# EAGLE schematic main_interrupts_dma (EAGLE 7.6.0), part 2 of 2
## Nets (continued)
Unconnected: IC1.1(CLR) IC1.11(CLK) IC2.1(A:G) IC2.2(A:A1) IC2.4(A:A2) IC2.6(A:A3) IC2.8(A:A4) IC2.12(A:Y4) IC2.14(A:Y3) IC2.16(A:Y2) IC2.18(A:Y1) IC3.1(A:G) IC3.2(A:A1) IC3.4(A:A2) IC3.6(A:A3) IC3.8(A:A4) IC3.12(A:Y4) IC3.14(A:Y3) IC3.16(A:Y2) IC3.18(A:Y1) IC4.11(CLK) IC5.11(CLK) IC6.11(CLK) IC10.3(B:Y4) IC10.17(B:A4) IC11.3(B:Y4) IC11.5(B:Y3) IC11.7(B:Y2) IC11.9(B:Y1) IC11.11(B:A1) IC11.13(B:A2) IC11.15(B:A3) IC11.17(B:A4) IC11.19(B:G) IC12.3(B:Y4) IC12.5(B:Y3) IC12.7(B:Y2) IC12.9(B:Y1) IC12.11(B:A1) IC12.13(B:A2) IC12.15(B:A3) IC12.17(B:A4) IC12.19(B:G) IC13.3(B:Y4) IC13.5(B:Y3) IC13.7(B:Y2) IC13.9(B:Y1) IC13.11(B:A1) IC13.13(B:A2) IC13.15(B:A3) IC13.17(B:A4) IC13.19(B:G) IC14.14(A=B) IC14.15(P) IC14.17(G) IC15.14(A=B) IC15.15(P) IC15.17(G) IC16.11(CLK) IC17.11(CLK) IC18.1(A:I0) IC18.2(A:I1) IC18.3(A:O) IC18.8(C:O) IC18.9(C:I0) IC18.10(C:I1) IC18.11(D:O) IC18.12(D:I0) IC18.13(D:I1) IC19.2(A:A1) IC19.4(A:A2) IC19.6(A:A3) IC19.8(A:A4) IC19.11(B:A1) IC19.13(B:A2) IC19.15(B:A3) IC19.17(B:A4) IC20.11(CLK) IC21.11(CLK) IC24.1(A:G) IC24.2(A:A1) IC24.4(A:A2) IC24.6(A:A3) IC24.8(A:A4) IC24.12(A:Y4) IC24.14(A:Y3) IC24.16(A:Y2) IC24.18(A:Y1) IC24.19(B:G) IC25.1(A:G) IC25.2(A:A1) IC25.4(A:A2) IC25.6(A:A3) IC25.8(A:A4) IC25.12(A:Y4) IC25.14(A:Y3) IC25.16(A:Y2) IC25.18(A:Y1) IC25.19(B:G) IC26.1(A:G) IC26.2(A:A1) IC26.4(A:A2) IC26.6(A:A3) IC26.8(A:A4) IC26.12(A:Y4) IC26.14(A:Y3) IC26.16(A:Y2) IC26.18(A:Y1) IC26.19(B:G) IC27.1(A:G) IC27.2(A:A1) IC27.4(A:A2) IC27.6(A:A3) IC27.8(A:A4) IC27.12(A:Y4) IC27.14(A:Y3) IC27.16(A:Y2) IC27.18(A:Y1) IC27.19(B:G) IC28.1(A:G) IC28.2(A:A1) IC28.4(A:A2) IC28.6(A:A3) IC28.8(A:A4) IC28.12(A:Y4) IC28.14(A:Y3) IC28.16(A:Y2) IC28.18(A:Y1) IC29.1(A:G) IC29.2(A:A1) IC29.4(A:A2) IC29.6(A:A3) IC29.8(A:A4) IC29.12(A:Y4) IC29.14(A:Y3) IC29.16(A:Y2) IC29.18(A:Y1) IC30.3(B:Y4) IC30.5(B:Y3) IC30.7(B:Y2) IC30.9(B:Y1) IC30.11(B:A1) IC30.13(B:A2) IC30.15(B:A3) IC30.17(B:A4) IC30.19(B:G) IC31.3(B:Y4) IC31.5(B:Y3) IC31.7(B:Y2) IC31.9(B:Y1) IC31.11(B:A1) IC31.13(B:A2) IC31.15(B:A3) IC31.17(B:A4) IC31.19(B:G) IC32.17(D7) IC32.18(D8) IC33.16(Q7) IC33.19(Q8) IC34.1(1G) IC34.15(2G) IC35.1(1G) IC35.15(2G) IC36.1(1G) IC36.15(2G) IC37.1(1G) IC37.15(2G) IC38.1(1G) IC38.10(2C0) IC38.15(2G) IC39.4(B:I0) IC39.5(B:I1) IC39.6(B:O) IC39.8(C:O) IC39.9(C:I0) IC39.10(C:I1) IC39.11(D:O) IC39.12(D:I0) IC39.13(D:I1) IC40.1(1G) IC40.15(2G) IC41.1(1G) IC41.15(2G) IC42.1(A:I) IC42.2(A:O) IC42.5(C:I) IC42.6(C:O) IC42.8(D:O) IC42.9(D:I) IC42.10(E:O) IC42.11(E:I) IC42.12(F:O) IC42.13(F:I) IC43.1(A:I) IC43.2(A:O) IC43.5(C:I) IC43.6(C:O) IC43.8(D:O) IC43.9(D:I) IC43.10(E:O) IC43.11(E:I) IC43.12(F:O) IC43.13(F:I) IC44.1(A:CLR) IC44.4(A:PRE) IC44.6(A:!Q) IC44.8(B:!Q) IC44.9(B:Q) IC44.10(B:PRE) IC44.11(B:CLK) IC44.12(B:D) IC44.13(B:CLR) IC45.1(A:I) IC45.2(A:O) IC45.5(C:I) IC45.6(C:O) IC45.8(D:O) IC45.9(D:I) IC45.10(E:O) IC45.11(E:I) IC45.12(F:O) IC45.13(F:I) IC46.1(G) IC46.11(CLK) IC46.12(5Q) IC46.15(6Q) IC46.16(7Q) IC46.19(8Q) IC47.1(!A!/B) IC47.15(G) IC48.11(CLK) IC49.1(A:I0) IC49.2(A:I1) IC49.3(A:O) IC49.4(B:I0) IC49.5(B:I1) IC49.6(B:O) IC49.8(C:O) IC49.9(C:I0) IC49.10(C:I1) IC53.9(C4) IC53.10(S4) IC53.13(S3) IC54.1(A:CLR) IC54.4(A:PRE) IC54.6(A:!Q) IC54.8(B:!Q) IC54.9(B:Q) IC54.10(B:PRE) IC54.11(B:CLK) IC54.12(B:D) IC54.13(B:CLR) IC55.3(B:I0) IC55.4(B:I1) IC55.5(B:I2) IC55.6(B:O) IC55.8(C:O) IC55.9(C:I0) IC55.10(C:I1) IC55.11(C:I2) IC56.2(B) IC56.9(2Y) IC56.10(2C0) IC56.11(2C1) IC56.12(2C2) IC56.13(2C3) IC56.14(A) IC57.5(C:I) IC57.6(C:O) IC57.8(D:O) IC57.9(D:I) IC57.10(E:O) IC57.11(E:I) IC57.12(F:O) IC57.13(F:I) IC58.4(B:I0) IC58.5(B:I1) IC58.6(B:O) IC58.8(C:O) IC58.9(C:I0) IC58.10(C:I1) IC58.11(D:O) IC58.12(D:I0) IC58.13(D:I1) IC59.15(G) IC60.1(CLR) IC60.2(Q1) IC60.5(Q2) IC60.6(Q3) IC60.9(Q4) IC60.12(Q5) IC60.15(Q6) IC60.16(Q7) IC60.19(Q8) IC61.1(CLR) IC61.2(Q1) IC61.5(Q2) IC61.6(Q3) IC61.9(Q4) IC61.12(Q5) IC61.15(Q6) IC61.16(Q7) IC61.19(Q8) IC62.1(CLR) IC62.2(Q1) IC62.5(Q2) IC62.6(Q3) IC62.9(Q4) IC62.12(Q5) IC62.15(Q6) IC62.16(Q7) IC62.19(Q8) IC63.11(CLK) IC64.8(B:O) IC64.9(B:I0) IC64.10(B:I1) IC64.12(B:I2) IC64.13(B:I3) IC65.3(B:I) IC65.4(B:O) IC65.5(C:I) IC65.6(C:O) IC65.8(D:O) IC65.9(D:I) IC65.10(E:O) IC65.11(E:I) IC65.12(F:O) IC65.13(F:I) IC66.4(B:I0) IC66.5(B:I1) IC66.6(B:O) IC66.8(C:O) IC66.9(C:I0) IC66.10(C:I1) IC66.11(D:O) IC66.12(D:I0) IC66.13(D:I1) IC67.1(A:I0) IC67.2(A:I1) IC67.3(A:O) IC67.8(C:O) IC67.9(C:I0) IC67.10(C:I1) IC67.11(D:O) IC67.12(D:I0) IC67.13(D:I1) IC68.4(B:I0) IC68.5(B:I1) IC68.6(B:O) IC68.8(C:O) IC68.9(C:I0) IC68.10(C:I1) IC68.11(D:O) IC68.12(D:I0) IC68.13(D:I1) IC69.4(B:I0) IC69.5(B:I1) IC69.6(B:O) IC69.8(C:O) IC69.9(C:I0) IC69.10(C:I1) IC69.11(D:O) IC69.12(D:I0) IC69.13(D:I1) IC70.1(A:G) IC70.2(A:A1) IC70.4(A:A2) IC70.6(A:A3) IC70.8(A:A4) IC70.12(A:Y4) IC70.14(A:Y3) IC70.16(A:Y2) IC70.18(A:Y1) IC71.1(A:G) IC71.2(A:A1) IC71.4(A:A2) IC71.6(A:A3) IC71.8(A:A4) IC71.12(A:Y4) IC71.14(A:Y3) IC71.16(A:Y2) IC71.18(A:Y1) IC72.1(A:I0) IC72.2(A:I1) IC72.3(A:O) IC72.8(C:O) IC72.9(C:I0) IC72.10(C:I1) IC72.11(D:O) IC72.12(D:I0) IC72.13(D:I1) IC73.5(2A) IC73.6(2B) IC73.7(2Y) IC73.9(3Y) IC73.10(3B) IC73.11(3A) IC73.12(4Y) IC73.13(4B) IC73.14(4A) IC73.15(G) IC74.1(A:I0) IC74.2(A:I1) IC74.3(A:O) IC74.8(C:O) IC74.9(C:I0) IC74.10(C:I1) IC74.11(D:O) IC74.12(D:I0) IC74.13(D:I1) IC75.2(Q1) IC75.5(Q2) IC75.6(Q3) IC75.9(Q4) IC75.12(Q5) IC75.15(Q6) IC80.1(A:I0) IC80.2(A:I1) IC80.3(A:O) IC80.8(C:O) IC80.9(C:I0) IC80.10(C:I1) IC80.11(D:O) IC80.12(D:I0) IC80.13(D:I1) IC81.1(A:I0) IC81.2(A:I1) IC81.3(A:O) IC81.8(C:O) IC81.9(C:I0) IC81.10(C:I1) IC81.11(D:O) IC81.12(D:I0) IC81.13(D:I1) IC82.3(B:Y4) IC82.5(B:Y3) IC82.7(B:Y2) IC82.9(B:Y1) IC82.11(B:A1) IC82.13(B:A2) IC82.15(B:A3) IC82.17(B:A4) IC82.19(B:G) IC83.3(B:Y4) IC83.5(B:Y3) IC83.7(B:Y2) IC83.9(B:Y1) IC83.11(B:A1) IC83.13(B:A2) IC83.15(B:A3) IC83.17(B:A4) IC83.19(B:G) IC84.3(B:Y4) IC84.5(B:Y3) IC84.7(B:Y2) IC84.9(B:Y1) IC84.11(B:A1) IC84.13(B:A2) IC84.15(B:A3) IC84.17(B:A4) IC84.19(B:G) IC85.3(B:Y4) IC85.5(B:Y3) IC85.7(B:Y2) IC85.9(B:Y1) IC85.11(B:A1) IC85.13(B:A2) IC85.15(B:A3) IC85.17(B:A4) IC85.19(B:G) IC86.11(CLK) IC87.2(A:S1) IC87.5(C:R) IC87.6(C:S) IC87.7(C:Q) IC87.9(B:Q) IC87.10(B:R) IC87.11(B:S1) IC87.12(B:S2) IC87.13(D:Q) IC87.14(D:R) IC87.15(D:S) IC88.11(CLK) IC89.3(B:Y4) IC89.5(B:Y3) IC89.7(B:Y2) IC89.9(B:Y1) IC89.11(B:A1) IC89.13(B:A2) IC89.15(B:A3) IC89.17(B:A4) IC89.19(B:G) IC90.3(B:Y4) IC90.5(B:Y3) IC90.7(B:Y2) IC90.9(B:Y1) IC90.11(B:A1) IC90.13(B:A2) IC90.15(B:A3) IC90.17(B:A4) IC90.19(B:G) IC91.3(B:Y4) IC91.5(B:Y3) IC91.7(B:Y2) IC91.9(B:Y1) IC91.11(B:A1) IC91.13(B:A2) IC91.15(B:A3) IC91.17(B:A4) IC91.19(B:G) IC92.3(B:Y4) IC92.5(B:Y3) IC92.7(B:Y2) IC92.9(B:Y1) IC92.11(B:A1) IC92.13(B:A2) IC92.15(B:A3) IC92.17(B:A4) IC92.19(B:G) IC93.11(CLK) IC94.11(CLK) IC95.3(B:Y4) IC95.5(B:Y3) IC95.7(B:Y2) IC95.9(B:Y1) IC95.11(B:A1) IC95.13(B:A2) IC95.15(B:A3) IC95.17(B:A4) IC95.19(B:G) IC96.3(B:Y4) IC96.5(B:Y3) IC96.7(B:Y2) IC96.9(B:Y1) IC96.11(B:A1) IC96.13(B:A2) IC96.15(B:A3) IC96.17(B:A4) IC96.19(B:G) IC97.3(B:Y4) IC97.5(B:Y3) IC97.7(B:Y2) IC97.9(B:Y1) IC97.11(B:A1) IC97.13(B:A2) IC97.15(B:A3) IC97.17(B:A4) IC97.19(B:G) IC98.1(CLR) IC98.11(CLK) IC99.11(CLK) IC100.1(CLR) IC100.11(CLK) IC100.18(D8) IC101.1(CLR) IC101.11(CLK) IC101.18(D8) IC102.1(A:G) IC102.2(A:A1) IC102.4(A:A2) IC102.6(A:A3) IC102.8(A:A4) IC102.12(A:Y4) IC102.14(A:Y3) IC102.16(A:Y2) IC102.18(A:Y1) IC103.11(CLK) IC104.11(CLK) IC105.1(A:G) IC105.2(A:A1) IC105.4(A:A2) IC105.6(A:A3) IC105.8(A:A4) IC105.12(A:Y4) IC105.14(A:Y3) IC105.16(A:Y2) IC105.18(A:Y1) IC106.1(A:G) IC106.2(A:A1) IC106.4(A:A2) IC106.6(A:A3) IC106.8(A:A4) IC106.12(A:Y4) IC106.14(A:Y3) IC106.16(A:Y2) IC106.18(A:Y1) IC107.1(A:G) IC107.2(A:A1) IC107.4(A:A2) IC107.6(A:A3) IC107.8(A:A4) IC107.12(A:Y4) IC107.14(A:Y3) IC107.16(A:Y2) IC107.18(A:Y1) IC108.1(A:G) IC108.2(A:A1) IC108.4(A:A2) IC108.6(A:A3) IC108.8(A:A4) IC108.12(A:Y4) IC108.14(A:Y3) IC108.16(A:Y2) IC108.18(A:Y1) IC109.1(A:G) IC109.2(A:A1) IC109.4(A:A2) IC109.6(A:A3) IC109.8(A:A4) IC109.12(A:Y4) IC109.14(A:Y3) IC109.16(A:Y2) IC109.18(A:Y1) IC110.1(A:G) IC110.2(A:A1) IC110.4(A:A2) IC110.6(A:A3) IC110.8(A:A4) IC110.12(A:Y4) IC110.14(A:Y3) IC110.16(A:Y2) IC110.18(A:Y1) IC111.1(A:G) IC111.2(A:A1) IC111.4(A:A2) IC111.6(A:A3) IC111.8(A:A4) IC111.12(A:Y4) IC111.14(A:Y3) IC111.16(A:Y2) IC111.18(A:Y1) IC112.1(A:G) IC112.2(A:A1) IC112.4(A:A2) IC112.6(A:A3) IC112.8(A:A4) IC112.12(A:Y4) IC112.14(A:Y3) IC112.16(A:Y2) IC112.18(A:Y1) IC113.1(A:G) IC113.2(A:A1) IC113.4(A:A2) IC113.6(A:A3) IC113.8(A:A4) IC113.12(A:Y4) IC113.14(A:Y3) IC113.16(A:Y2) IC113.18(A:Y1) IC114.1(A:G) IC114.2(A:A1) IC114.4(A:A2) IC114.6(A:A3) IC114.8(A:A4) IC114.12(A:Y4) IC114.14(A:Y3) IC114.16(A:Y2) IC114.18(A:Y1) IC115.1(A:G) IC115.2(A:A1) IC115.4(A:A2) IC115.6(A:A3) IC115.8(A:A4) IC115.12(A:Y4) IC115.14(A:Y3) IC115.16(A:Y2) IC115.18(A:Y1) IC116.1(A:G) IC116.2(A:A1) IC116.4(A:A2) IC116.6(A:A3) IC116.8(A:A4) IC116.12(A:Y4) IC116.14(A:Y3) IC116.16(A:Y2) IC116.18(A:Y1) IC117.1(A:G) IC117.2(A:A1) IC117.4(A:A2) IC117.6(A:A3) IC117.8(A:A4) IC117.12(A:Y4) IC117.14(A:Y3) IC117.16(A:Y2) IC117.18(A:Y1) IC118.1(G1) IC118.11(Y8) IC118.12(Y7) IC118.19(G2) IC119.3(B:Y4) IC119.5(B:Y3) IC119.7(B:Y2) IC119.9(B:Y1) IC119.11(B:A1) IC119.13(B:A2) IC119.15(B:A3) IC119.17(B:A4) IC119.19(B:G) IC120.11(CLK) IC121.11(CLK) IC122.3(B:Y4) IC122.5(B:Y3) IC122.7(B:Y2) IC122.9(B:Y1) IC122.11(B:A1) IC122.13(B:A2) IC122.15(B:A3) IC122.17(B:A4) IC122.19(B:G) IC123.3(B:Y4) IC123.5(B:Y3) IC123.7(B:Y2) IC123.9(B:Y1) IC123.11(B:A1) IC123.13(B:A2) IC123.15(B:A3) IC123.17(B:A4) IC123.19(B:G) IC124.3(B:Y4) IC124.5(B:Y3) IC124.7(B:Y2) IC124.9(B:Y1) IC124.11(B:A1) IC124.13(B:A2) IC124.15(B:A3) IC124.17(B:A4) IC124.19(B:G) IC125.3(B:Y4) IC125.5(B:Y3) IC125.7(B:Y2) IC125.9(B:Y1) IC125.11(B:A1) IC125.13(B:A2) IC125.15(B:A3) IC125.17(B:A4) IC125.19(B:G) IC126.11(CLK) IC126.12(5Q) IC126.13(5D) IC126.14(6D) IC126.15(6Q) IC126.16(7Q) IC126.17(7D) IC126.18(8D) IC126.19(8Q) IC127.1(A:G) IC127.2(A:A1) IC127.4(A:A2) IC127.6(A:A3) IC127.8(A:A4) IC127.12(A:Y4) IC127.14(A:Y3) IC127.16(A:Y2) IC127.18(A:Y1) IC128.11(CLK) IC129.2(A:A1) IC129.4(A:A2) IC129.6(A:A3) IC129.8(A:A4) IC129.11(B:A1) IC129.13(B:A2) IC129.15(B:A3) IC129.17(B:A4) IC130.1(A:I0) IC130.2(A:I1) IC130.3(A:O) IC130.8(C:O) IC130.9(C:I0) IC130.10(C:I1) IC130.11(D:O) IC130.12(D:I0) IC130.13(D:I1) IC131.8(B:O) IC131.9(B:I0) IC131.10(B:I1) IC131.12(B:I2) IC131.13(B:I3) IC132.3(B:I) IC132.4(B:O) IC132.5(C:I) IC132.6(C:O) IC132.8(D:O) IC132.9(D:I) IC132.10(E:O) IC132.11(E:I) IC132.12(F:O) IC132.13(F:I) IC133.3(A:O) IC133.4(B:I0) IC133.5(B:I1) IC133.6(B:O) IC133.8(C:O) IC133.9(C:I0) IC133.10(C:I1) IC133.11(D:O) IC133.12(D:I0) IC133.13(D:I1) IC138.4(B:I0) IC138.5(B:I1) IC138.6(B:O) IC138.8(C:O) IC138.9(C:I0) IC138.10(C:I1) IC138.11(D:O) IC138.12(D:I0) IC138.13(D:I1) IC139.4(Q2) IC139.5(Q3) IC139.6(Q4) IC139.11(D4) IC139.12(D3) IC139.13(D2) IC140.1(G1) IC140.19(G2) IC141.3(B:I) IC141.4(B:O) IC141.5(C:I) IC141.6(C:O) IC141.8(D:O) IC141.9(D:I) IC141.10(E:O) IC141.11(E:I) IC141.12(F:O) IC141.13(F:I) IC142.1(1G) IC142.15(2G) IC143.4(B:I0) IC143.5(B:I1) IC143.6(B:O) IC143.8(C:O) IC143.9(C:I0) IC143.10(C:I1) IC143.11(D:O) IC143.12(D:I0) IC143.13(D:I1) IC144.1(CLR) IC144.11(CLK) IC144.18(D8) IC145.1(A:G) IC145.2(A:A1) IC145.4(A:A2) IC145.6(A:A3) IC145.8(A:A4) IC145.12(A:Y4) IC145.14(A:Y3) IC145.16(A:Y2) IC145.18(A:Y1) IC146.1(A:G) IC146.2(A:A1) IC146.4(A:A2) IC146.6(A:A3) IC146.8(A:A4) IC146.12(A:Y4) IC146.14(A:Y3) IC146.16(A:Y2) IC146.18(A:Y1) IC147.10 IC147.11 IC148.1(A:I0) IC148.2(A:I1) IC148.3(A:O) IC148.4(B:I0) IC148.5(B:I1) IC148.6(B:O) IC148.8(C:O) IC148.9(C:I0) IC148.10(C:I1) IC149.1(A:I0) IC149.2(A:I1) IC149.3(A:O) IC149.4(B:I0) IC149.5(B:I1) IC149.6(B:O) IC150.3(B:I) IC150.4(B:O) IC150.5(C:I) IC150.6(C:O) IC150.8(D:O) IC150.9(D:I) IC150.10(E:O) IC150.11(E:I) IC150.12(F:O) IC150.13(F:I) IC151.3(B:I) IC151.4(B:O) IC151.5(C:I) IC151.6(C:O) IC151.8(D:O) IC151.9(D:I) IC151.10(E:O) IC151.11(E:I) IC151.12(F:O) IC151.13(F:I) IC152.1(A:G) IC152.2(A:A1) IC152.4(A:A2) IC152.6(A:A3) IC152.8(A:A4) IC152.12(A:Y4) IC152.14(A:Y3) IC152.15(B:A3) IC152.16(A:Y2) IC152.17(B:A4) IC152.18(A:Y1) IC153.1(A:G) IC153.2(A:A1) IC153.4(A:A2) IC153.6(A:A3) IC153.8(A:A4) IC153.12(A:Y4) IC153.14(A:Y3) IC153.16(A:Y2) IC153.18(A:Y1) IC154.1(A:G) IC154.2(A:A1) IC154.4(A:A2) IC154.6(A:A3) IC154.8(A:A4) IC154.12(A:Y4) IC154.14(A:Y3) IC154.16(A:Y2) IC154.18(A:Y1) IC155.1(A:I) IC155.2(A:O) IC155.5(C:I) IC155.6(C:O) IC155.8(D:O) IC155.9(D:I) IC155.10(E:O) IC155.11(E:I) IC155.12(F:O) IC155.13(F:I) IC157.3(B:I) IC157.4(B:O) IC157.5(C:I) IC157.6(C:O) IC157.8(D:O) IC157.9(D:I) IC157.10(E:O) IC157.11(E:I) IC157.12(F:O) IC157.13(F:I) IC158.3(B:I) IC158.4(B:O) IC158.5(C:I) IC158.6(C:O) IC158.8(D:O) IC158.9(D:I) IC158.10(E:O) IC158.11(E:I) IC158.12(F:O) IC158.13(F:I) IC159.1(CLR) IC159.16(Q7) IC159.19(Q8) IC161.4(A:PRE) IC161.6(A:!Q) IC161.8(B:!Q) IC161.9(B:Q) IC161.10(B:PRE) IC161.11(B:CLK) IC161.12(B:D) IC161.13(B:CLR) IC162.4(A:PRE) IC162.6(A:!Q) IC162.8(B:!Q) IC162.9(B:Q) IC162.10(B:PRE) IC162.11(B:CLK) IC162.12(B:D) IC162.13(B:CLR) IC163.3(A:CLK) IC163.4(A:PRE) IC163.6(A:!Q) IC163.8(B:!Q) IC163.9(B:Q) IC163.10(B:PRE) IC163.11(B:CLK) IC163.12(B:D) IC163.13(B:CLR) IC167.4(B:I0) IC167.5(B:I1) IC167.6(B:O) IC167.8(C:O) IC167.9(C:I0) IC167.10(C:I1) IC167.11(D:O) IC167.12(D:I0) IC167.13(D:I1) IC168.3(A:CLK) IC168.4(A:PRE) IC168.6(A:!Q) IC168.8(B:!Q) IC168.9(B:Q) IC168.10(B:PRE) IC168.11(B:CLK) IC168.12(B:D) IC168.13(B:CLR) IC169.4(A:PRE) IC169.6(A:!Q) IC169.8(B:!Q) IC169.9(B:Q) IC169.10(B:PRE) IC169.11(B:CLK) IC169.12(B:D) IC169.13(B:CLR) IC170.1(A:I0) IC170.2(A:I1) IC170.3(A:O) IC170.8(C:O) IC170.9(C:I0) IC170.10(C:I1) IC170.11(D:O) IC170.12(D:I0) IC170.13(D:I1) IC174.4(B:I0) IC174.5(B:I1) IC174.6(B:O) IC174.8(C:O) IC174.9(C:I0) IC174.10(C:I1) IC174.11(D:O) IC174.12(D:I0) IC174.13(D:I1) IC175.3(A:CLK) IC175.4(A:PRE) IC175.6(A:!Q) IC175.8(B:!Q) IC175.9(B:Q) IC175.10(B:PRE) IC175.11(B:CLK) IC175.12(B:D) IC175.13(B:CLR) IC179.4(B:I0) IC179.5(B:I1) IC179.6(B:O) IC179.8(C:O) IC179.9(C:I0) IC179.10(C:I1) IC179.11(D:O) IC179.12(D:I0) IC179.13(D:I1) IC183.1(A:I) IC183.2(A:O) IC183.5(C:I) IC183.6(C:O) IC183.8(D:O) IC183.9(D:I) IC183.10(E:O) IC183.11(E:I) IC183.12(F:O) IC183.13(F:I) IC185.4(B:I0) IC185.5(B:I1) IC185.6(B:O) IC185.8(C:O) IC185.9(C:I0) IC185.10(C:I1) IC185.11(D:O) IC185.12(D:I0) IC185.13(D:I1) IC190.11(CLK) IC191.1(A:G) IC191.2(A:A1) IC191.4(A:A2) IC191.6(A:A3) IC191.8(A:A4) IC191.12(A:Y4) IC191.14(A:Y3) IC191.16(A:Y2) IC191.18(A:Y1) IC192.1(A:G) IC192.2(A:A1) IC192.4(A:A2) IC192.6(A:A3) IC192.8(A:A4) IC192.12(A:Y4) IC192.14(A:Y3) IC192.16(A:Y2) IC192.18(A:Y1) IC193.1(A:G) IC193.2(A:A1) IC193.4(A:A2) IC193.6(A:A3) IC193.8(A:A4) IC193.12(A:Y4) IC193.14(A:Y3) IC193.16(A:Y2) IC193.18(A:Y1) IC194.1(A:G) IC194.2(A:A1) IC194.4(A:A2) IC194.6(A:A3) IC194.8(A:A4) IC194.12(A:Y4) IC194.14(A:Y3) IC194.16(A:Y2) IC194.18(A:Y1) IC195.1(A:G) IC195.2(A:A1) IC195.4(A:A2) IC195.6(A:A3) IC195.8(A:A4) IC195.12(A:Y4) IC195.14(A:Y3) IC195.16(A:Y2) IC195.18(A:Y1) IC196.1(A:G) IC196.2(A:A1) IC196.4(A:A2) IC196.6(A:A3) IC196.8(A:A4) IC196.12(A:Y4) IC196.14(A:Y3) IC196.16(A:Y2) IC196.18(A:Y1) IC197.4(B:I0) IC197.6(B:O) IC197.8(B:I1) IC197.9(B:I2) IC197.10(B:I3) IC197.11(B:I4) IC198.3(B:I) IC198.4(B:O) IC198.5(C:I) IC198.6(C:O) IC198.8(D:O) IC198.9(D:I) IC198.10(E:O) IC198.11(E:I) IC198.12(F:O) IC198.13(F:I) IC199.4(B:I0) IC199.6(B:O) IC199.8(B:I1) IC199.9(B:I2) IC199.10(B:I3) IC199.11(B:I4) IC200.11(CLK) IC201.3(B:Y4) IC201.5(B:Y3) IC201.7(B:Y2) IC201.9(B:Y1) IC201.11(B:A1) IC201.13(B:A2) IC201.15(B:A3) IC201.17(B:A4) IC201.19(B:G) IC202.3(B:Y4) IC202.5(B:Y3) IC202.7(B:Y2) IC202.9(B:Y1) IC202.11(B:A1) IC202.13(B:A2) IC202.15(B:A3) IC202.17(B:A4) IC202.19(B:G) IC203.3(B:Y4) IC203.5(B:Y3) IC203.7(B:Y2) IC203.9(B:Y1) IC203.11(B:A1) IC203.12(A:Y4) IC203.13(B:A2) IC203.15(B:A3) IC203.17(B:A4) IC203.19(B:G) IC204.3(B:Y4) IC204.5(B:Y3) IC204.7(B:Y2) IC204.9(B:Y1) IC204.11(B:A1) IC204.13(B:A2) IC204.15(B:A3) IC204.17(B:A4) IC204.19(B:G) IC205.3(B:Y4) IC205.5(B:Y3) IC205.7(B:Y2) IC205.9(B:Y1) IC205.11(B:A1) IC205.13(B:A2) IC205.15(B:A3) IC205.17(B:A4) IC205.19(B:G) IC206.3(B:Y4) IC206.5(B:Y3) IC206.7(B:Y2) IC206.9(B:Y1) IC206.11(B:A1) IC206.13(B:A2) IC206.15(B:A3) IC206.17(B:A4) IC206.19(B:G) IC207.3(B:Y4) IC207.5(B:Y3) IC207.7(B:Y2) IC207.9(B:Y1) IC207.11(B:A1) IC207.13(B:A2) IC207.15(B:A3) IC207.17(B:A4) IC207.19(B:G) IC208.3(B:Y4) IC208.5(B:Y3) IC208.7(B:Y2) IC208.9(B:Y1) IC208.11(B:A1) IC208.13(B:A2) IC208.15(B:A3) IC208.17(B:A4) IC208.19(B:G) IC209.11(CLK) IC210.11(CLK) IC211.3(B:Y4) IC211.5(B:Y3) IC211.7(B:Y2) IC211.9(B:Y1) IC211.11(B:A1) IC211.13(B:A2) IC211.15(B:A3) IC211.17(B:A4) IC211.19(B:G) IC212.3(B:Y4) IC212.5(B:Y3) IC212.7(B:Y2) IC212.9(B:Y1) IC212.11(B:A1) IC212.13(B:A2) IC212.15(B:A3) IC212.17(B:A4) IC212.19(B:G) IC213.3(B:Y4) IC213.5(B:Y3) IC213.7(B:Y2) IC213.9(B:Y1) IC213.11(B:A1) IC213.13(B:A2) IC213.15(B:A3) IC213.17(B:A4) IC213.19(B:G) IC214.3(B:Y4) IC214.5(B:Y3) IC214.7(B:Y2) IC214.9(B:Y1) IC214.11(B:A1) IC214.13(B:A2) IC214.15(B:A3) IC214.17(B:A4) IC214.19(B:G) IC215.11(CLK) IC216.11(CLK) IC217.3(B:Y4) IC217.5(B:Y3) IC217.7(B:Y2) IC217.9(B:Y1) IC217.11(B:A1) IC217.13(B:A2) IC217.15(B:A3) IC217.17(B:A4) IC217.19(B:G) IC218.3(B:Y4) IC218.5(B:Y3) IC218.7(B:Y2) IC218.9(B:Y1) IC218.11(B:A1) IC218.13(B:A2) IC218.15(B:A3) IC218.17(B:A4) IC218.19(B:G) IC219.3(B:Y4) IC219.5(B:Y3) IC219.7(B:Y2) IC219.9(B:Y1) IC219.11(B:A1) IC219.13(B:A2) IC219.15(B:A3) IC219.17(B:A4) IC219.19(B:G) IC220.3(B:Y4) IC220.5(B:Y3) IC220.7(B:Y2) IC220.9(B:Y1) IC220.11(B:A1) IC220.13(B:A2) IC220.15(B:A3) IC220.17(B:A4) IC220.19(B:G) IC221.3(A:CLK) IC221.4(A:PRE) IC221.6(A:!Q) IC221.8(B:!Q) IC221.9(B:Q) IC221.10(B:PRE) IC221.11(B:CLK) IC221.12(B:D) IC221.13(B:CLR) IC222.15(Y0) S2.1(O) SW3.8 U$1.28(VCC) U$2.28(VCC) U$3.28(VCC) U$4.28(VCC) U$5.28(VCC) U$6.28(VCC) U$7.28(VCC) U$8.28(VCC) U$9.28(VCC) U$10.1(A14) U$10.2(A12) U$10.3(A7) U$10.4(A6) U$10.5(A5) U$10.6(A4) U$10.7(A3) U$10.8(A2) U$10.9(A1) U$10.10(A0) U$10.14(GND) U$10.20(/CE) U$10.21(A10) U$10.22(/OE) U$10.23(A11) U$10.24(A9) U$10.25(A8) U$10.26(A13) U$10.27(/WE) U$10.28(VCC) U$11.1(A14) U$11.2(A12) U$11.3(A7) U$11.4(A6) U$11.5(A5) U$11.6(A4) U$11.7(A3) U$11.8(A2) U$11.9(A1) U$11.10(A0) U$11.14(GND) U$11.20(/CE) U$11.21(A10) U$11.22(/OE) U$11.23(A11) U$11.24(A9) U$11.25(A8) U$11.26(A13) U$11.27(/WE) U$11.28(VCC) U$12.1(A14) U$12.2(A12) U$12.3(A7) U$12.4(A6) U$12.5(A5) U$12.6(A4) U$12.7(A3) U$12.8(A2) U$12.9(A1) U$12.10(A0) U$12.14(GND) U$12.20(/CE) U$12.21(A10) U$12.22(/OE) U$12.23(A11) U$12.24(A9) U$12.25(A8) U$12.26(A13) U$12.27(/WE) U$12.28(VCC)

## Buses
XBUS[0..7]
ZBUS[0..7]
YBUS[0..7]
B$4
AD[0..15]
MDR_IN_BUS[0..7]
U_AD[0..13]
DATA[0..7]
U_AD_BUFF[0..13]
Z_BUS[0..7]
CTRL_BUS[0..2]

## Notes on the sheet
- SYNCHRONIZED INTERRUPT INPUTS
- TDR0
- IMMX | TDR1
- FROM MICROCODE
- SINGLE STEP CLOCK
- SINGLE STEP CLOCK
- fast clock
- slow clock
- TDR2
- TDR3
- U-ADDRESS MUX
- IR
- PCL
- U-CODE ROMS
- U-ADDRESS
- U-CODE FF'S
- Z BUS
- A
- ADDRESS & DATA BUSES NEED PULL DOWN RESISTORS 
  BECAUSE THE CPU BUS OUTPUTS HAVE 
  244'S WHICH ARE CLOSED MOST OF THE TIME.
- PCH
- LOW | ADDRESS BUS
- MARL
- LOW
- ADDER
- HIGH
- B | SPL
- ADDER | MAR is tri-stated when in programming mode.
- programming mode signal goes here to tell MAR to go tristate | MARH
- SPH
- AUX FLAGS
- C
- U-CODE FF'S
- MASK_4.5
- MASK_5.5 | BPL
- HIGH
- D
- MASK_FLAGS
- BPH
- U-ADDRESS MUX
- Z BUS
- U-ADDR MUX LOGIC
- CarryIn_Mux0
- CarryIn_Mux1
- CARRY IN MUX
- CONDITION SOURCE
  PROGRAMMER'S FLAGS 
  OR
  U_CODE FLAGS
- DATA BUS
- BUS GOING INTO MDR INPUTS
- MDR_Mux | MDR MUX | /MDR_X_Out | X BUS BUFFER
- IMMX
- BUS GOING INTO MDR INPUTS
- X BUS
- MDR MUX
- MDR
- IMMY | MDR MUX
- ALU
- MDR_Y_Out | Y BUS BUFFER
- alu_mode removed. OF is undefined if alu in logic mode anyway. | alu_op == add
- U_FLAGS
- DATA BUS
- DATA BUS
- /MDR_DataB_Out
- ALU_OP == SUB
- TDR0
- IMMY
- FROM MICROCODE
- TDR1
- TDR2
- TDR3
- THESE TDR'S ARE THE SAME ONES AS ARE CONNECTED TO THE X BUS

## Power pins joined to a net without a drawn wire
GND: IC1.10(GND) IC2.10(P:GND) IC3.10(P:GND) IC4.10(GND) IC5.10(GND) IC6.10(GND) IC7.10(GND) IC8.10(GND) IC9.10(P:GND) IC10.10(P:GND) IC11.10(P:GND) IC12.10(P:GND) IC13.10(P:GND) IC14.12(GND) IC15.12(GND) IC16.10(GND) IC17.10(GND) IC18.7(P:GND) IC19.10(P:GND) IC20.10(GND) IC21.10(GND) IC22.8(GND) IC23.8(GND) IC24.10(P:GND) IC25.10(P:GND) IC26.10(P:GND) IC27.10(P:GND) IC28.10(P:GND) IC29.10(P:GND) IC30.10(P:GND) IC31.10(P:GND) IC32.10(GND) IC33.10(GND) IC34.8(GND) IC35.8(GND) IC36.8(GND) IC37.8(GND) IC38.8(GND) IC39.7(P:GND) IC40.8(GND) IC41.8(GND) IC42.7(P:GND) IC43.7(P:GND) IC44.7(P:GND) IC45.7(P:GND) IC46.10(GND) IC47.8(GND) IC48.10(GND) IC49.7(P:GND) IC50.8(GND) IC51.8(GND) IC52.8(GND) IC53.8(GND) IC54.7(P:GND) IC55.7(P:GND) IC56.8(GND) IC57.7(P:GND) IC58.7(P:GND) IC59.8(GND) IC60.10(GND) IC61.10(GND) IC62.10(GND) IC63.10(GND) IC64.7(P:GND) IC65.7(P:GND) IC66.7(P:GND) IC67.7(P:GND) IC68.7(P:GND) IC69.7(P:GND) IC70.10(P:GND) IC71.10(P:GND) IC72.7(P:GND) IC73.8(GND) IC74.7(P:GND) IC75.10(GND) IC76.10(GND) IC77.10(GND) IC78.10(GND) IC79.10(GND) IC80.7(P:GND) IC81.7(P:GND) IC82.10(P:GND) IC83.10(P:GND) IC84.10(P:GND) IC85.10(P:GND) IC86.10(GND) IC87.8(P:GND) IC88.10(GND) IC89.10(P:GND) IC90.10(P:GND) IC91.10(P:GND) IC92.10(P:GND) IC93.10(GND) IC94.10(GND) IC95.10(P:GND) IC96.10(P:GND) IC97.10(P:GND) IC98.10(GND) IC99.10(GND) IC100.10(GND) IC101.10(GND) IC102.10(P:GND) IC103.10(GND) IC104.10(GND) IC105.10(P:GND) IC106.10(P:GND) IC107.10(P:GND) IC108.10(P:GND) IC109.10(P:GND) IC110.10(P:GND) IC111.10(P:GND) IC112.10(P:GND) IC113.10(P:GND) IC114.10(P:GND) IC115.10(P:GND) IC116.10(P:GND) IC117.10(P:GND) IC118.10(GND) IC119.10(P:GND) IC120.10(GND) IC121.10(GND) IC122.10(P:GND) IC123.10(P:GND) IC124.10(P:GND) IC125.10(P:GND) IC126.10(GND) IC127.10(P:GND) IC128.10(GND) IC129.10(P:GND) IC130.7(P:GND) IC131.7(P:GND) IC132.7(P:GND) IC133.7(P:GND) IC134.10(GND) IC135.10(GND) IC136.10(GND) IC137.10(GND) IC138.7(P:GND) IC139.8(GND) IC140.10(GND) IC141.7(P:GND) IC142.8(GND) IC143.7(P:GND) IC144.10(GND) IC145.10(P:GND) IC146.10(P:GND) IC147.8(GND) IC148.7(P:GND) IC149.7(P:GND) IC150.7(P:GND) IC151.7(P:GND) IC152.10(P:GND) IC153.10(P:GND) IC154.10(P:GND) IC155.7(P:GND) IC157.7(P:GND) IC158.7(P:GND) IC159.10(GND) IC161.7(P:GND) IC162.7(P:GND) IC163.7(P:GND) IC167.7(P:GND) IC168.7(P:GND) IC169.7(P:GND) IC170.7(P:GND) IC174.7(P:GND) IC175.7(P:GND) IC179.7(P:GND) IC183.7(P:GND) IC185.7(P:GND) IC190.10(GND) IC191.10(P:GND) IC192.10(P:GND) IC193.10(P:GND) IC194.10(P:GND) IC195.10(P:GND) IC196.10(P:GND) IC197.7(P:GND) IC198.7(P:GND) IC199.7(P:GND) IC200.10(GND) IC201.10(P:GND) IC202.10(P:GND) IC203.10(P:GND) IC204.10(P:GND) IC205.10(P:GND) IC206.10(P:GND) IC207.10(P:GND) IC208.10(P:GND) IC209.10(GND) IC210.10(GND) IC211.10(P:GND) IC212.10(P:GND) IC213.10(P:GND) IC214.10(P:GND) IC215.10(GND) IC216.10(GND) IC217.10(P:GND) IC218.10(P:GND) IC219.10(P:GND) IC220.10(P:GND) IC221.7(P:GND) IC222.8(GND)
VCC: IC1.20(VCC) IC2.20(P:VCC) IC3.20(P:VCC) IC4.20(VCC) IC5.20(VCC) IC6.20(VCC) IC7.20(VCC) IC8.20(VCC) IC9.20(P:VCC) IC10.20(P:VCC) IC11.20(P:VCC) IC12.20(P:VCC) IC13.20(P:VCC) IC14.24(VCC) IC15.24(VCC) IC16.20(VCC) IC17.20(VCC) IC18.14(P:VCC) IC19.20(P:VCC) IC20.20(VCC) IC21.20(VCC) IC22.16(VCC) IC23.16(VCC) IC24.20(P:VCC) IC25.20(P:VCC) IC26.20(P:VCC) IC27.20(P:VCC) IC28.20(P:VCC) IC29.20(P:VCC) IC30.20(P:VCC) IC31.20(P:VCC) IC32.20(VCC) IC33.20(VCC) IC34.16(VCC) IC35.16(VCC) IC36.16(VCC) IC37.16(VCC) IC38.16(VCC) IC39.14(P:VCC) IC40.16(VCC) IC41.16(VCC) IC42.14(P:VCC) IC43.14(P:VCC) IC44.14(P:VCC) IC45.14(P:VCC) IC46.20(VCC) IC47.16(VCC) IC48.20(VCC) IC49.14(P:VCC) IC50.16(VCC) IC51.16(VCC) IC52.16(VCC) IC53.16(VCC) IC54.14(P:VCC) IC55.14(P:VCC) IC56.16(VCC) IC57.14(P:VCC) IC58.14(P:VCC) IC59.16(VCC) IC60.20(VCC) IC61.20(VCC) IC62.20(VCC) IC63.20(VCC) IC64.14(P:VCC) IC65.14(P:VCC) IC66.14(P:VCC) IC67.14(P:VCC) IC68.14(P:VCC) IC69.14(P:VCC) IC70.20(P:VCC) IC71.20(P:VCC) IC72.14(P:VCC) IC73.16(VCC) IC74.14(P:VCC) IC75.20(VCC) IC76.20(VCC) IC77.20(VCC) IC78.20(VCC) IC79.20(VCC) IC80.14(P:VCC) IC81.14(P:VCC) IC82.20(P:VCC) IC83.20(P:VCC) IC84.20(P:VCC) IC85.20(P:VCC) IC86.20(VCC) IC87.16(P:VCC) IC88.20(VCC) IC89.20(P:VCC) IC90.20(P:VCC) IC91.20(P:VCC) IC92.20(P:VCC) IC93.20(VCC) IC94.20(VCC) IC95.20(P:VCC) IC96.20(P:VCC) IC97.20(P:VCC) IC98.20(VCC) IC99.20(VCC) IC100.20(VCC) IC101.20(VCC) IC102.20(P:VCC) IC103.20(VCC) IC104.20(VCC) IC105.20(P:VCC) IC106.20(P:VCC) IC107.20(P:VCC) IC108.20(P:VCC) IC109.20(P:VCC) IC110.20(P:VCC) IC111.20(P:VCC) IC112.20(P:VCC) IC113.20(P:VCC) IC114.20(P:VCC) IC115.20(P:VCC) IC116.20(P:VCC) IC117.20(P:VCC) IC118.20(VCC) IC119.20(P:VCC) IC120.20(VCC) IC121.20(VCC) IC122.20(P:VCC) IC123.20(P:VCC) IC124.20(P:VCC) IC125.20(P:VCC) IC126.20(VCC) IC127.20(P:VCC) IC128.20(VCC) IC129.20(P:VCC) IC130.14(P:VCC) IC131.14(P:VCC) IC132.14(P:VCC) IC133.14(P:VCC) IC134.20(VCC) IC135.20(VCC) IC136.20(VCC) IC137.20(VCC) IC138.14(P:VCC) IC139.16(VCC) IC140.20(VCC) IC141.14(P:VCC) IC142.16(VCC) IC143.14(P:VCC) IC144.20(VCC) IC145.20(P:VCC) IC146.20(P:VCC) IC147.16(VCC) IC148.14(P:VCC) IC149.14(P:VCC) IC150.14(P:VCC) IC151.14(P:VCC) IC152.20(P:VCC) IC153.20(P:VCC) IC154.20(P:VCC) IC155.14(P:VCC) IC157.14(P:VCC) IC158.14(P:VCC) IC159.20(VCC) IC161.14(P:VCC) IC162.14(P:VCC) IC163.14(P:VCC) IC167.14(P:VCC) IC168.14(P:VCC) IC169.14(P:VCC) IC170.14(P:VCC) IC174.14(P:VCC) IC175.14(P:VCC) IC179.14(P:VCC) IC183.14(P:VCC) IC185.14(P:VCC) IC190.20(VCC) IC191.20(P:VCC) IC192.20(P:VCC) IC193.20(P:VCC) IC194.20(P:VCC) IC195.20(P:VCC) IC196.20(P:VCC) IC197.14(P:VCC) IC198.14(P:VCC) IC199.14(P:VCC) IC200.20(VCC) IC201.20(P:VCC) IC202.20(P:VCC) IC203.20(P:VCC) IC204.20(P:VCC) IC205.20(P:VCC) IC206.20(P:VCC) IC207.20(P:VCC) IC208.20(P:VCC) IC209.20(VCC) IC210.20(VCC) IC211.20(P:VCC) IC212.20(P:VCC) IC213.20(P:VCC) IC214.20(P:VCC) IC215.20(VCC) IC216.20(VCC) IC217.20(P:VCC) IC218.20(P:VCC) IC219.20(P:VCC) IC220.20(P:VCC) IC221.14(P:VCC) IC222.16(VCC)

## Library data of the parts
IC1 IC4-IC8 IC16 IC17 IC20 IC21 IC32 IC33 IC48 IC60-IC63 IC75-IC79 IC86 IC88 IC93 IC94 IC98-IC101 IC103 IC104 IC120 IC121 IC134-IC137 IC144 IC159 IC200 IC209 IC210 IC215 IC216 = 74xx-us:74*273: Octal D type FLIP FLOP, clear
IC2 IC3 IC9-IC13 IC19 IC24-IC31 IC70 IC71 IC82-IC85 IC89-IC92 IC95-IC97 IC102 IC105-IC117 IC119 IC122-IC125 IC127 IC129 IC145 IC146 IC152-IC154 IC191-IC196 IC201-IC208 IC211-IC214 IC217-IC220 = 74xx-us:74*244: Octal BUFFER and LINE DRIVER, 3-state
IC14 IC15 = 74xx-us:74*181: ARITHMETIC LOGIC UNIT function generator
IC18 IC67 IC81 IC170 = 74xx-us:74*32: Quad 2-input OR gate
IC22 IC23 IC47 = 74xx-us:74*157: Quadruple 2-line to 1-line data SELECTOR/MULTIPLEXER
IC34-IC38 IC40 IC41 IC56 IC142 = 74xx-us:74*153: Dual 4-line to 1-line data SELECTOR/MULTIPLEXER
IC39 IC66 IC68 IC69 IC133 IC138 IC143 = 74xx-us:74*08: Quad 2-input AND gate
IC42 IC43 IC45 IC57 IC65 IC132 IC141 IC150 IC151 IC155 IC157 IC158 IC183 IC198 = 74xx-us:74*04: Hex INVERTER
IC44 IC54 IC161-IC163 IC168 IC169 IC175 IC221 = 74xx-us:74*74: Dual D type positive edge triggered FLIP FLOP, preset and clear
IC46 IC126 IC128 IC190 = 74xx-us:74*377: Octal D type FLIP FLOP, enable
IC49 IC148 IC149 IC167 IC174 IC179 IC185 = 74xx-us:74*00: Quad 2-input NAND gate
IC50-IC53 = 74xx-us:74*283: 4-bit binary FULL ADDER, fast carry
IC55 = 74xx-us:74*11: Triple 3-input AND gate
IC58 IC72 IC74 IC80 IC130 = 74xx-us:74*86: Quad 2-input EXCLUSIV-OR (XOR) gate
IC59 IC73 = 74xx-us:74*257: Quadruple 2-to 1 line data SELECTOR/MULTIPLEXER
IC64 IC131 = 74xx-us:74*20: Dual 4-input NAND gate
IC87 = 74xx-us:74*279: Quadruple S-R LATCH
IC118 IC140 = 74xx-us:74*541: Octal BUFFER and LINE DRIVER, 3-state
IC139 = 74xx-us:74*173: 4-bit D type REGISTER, 3-state
IC147 = 74xx-us:74*148: 10-line to 4-line and 8-line to 3-line PRIORITY ENCODER
IC197 IC199 = 74xx-us:74*260: Dual 5-input positive NOR gate
IC222 = 74xx-us:74*138: 3-line to 8-line DECODER/DEMULTIPLEXER
R1-R3 = rcl:R-US_: RESISTOR, American symbol
S1 S2 = switch:TL36PO: TINY SWITCH ON - ON Source: http://www2.produktinfo.conrad.com/datenblaetter/700000-724999/705152-da-01-de-Subminiaturschalter_TL_36YO.pdf
SW3 = special:SW-C10: SWITCH 10-step rotary switch
U$1-U$12 = atmel_28c:AT28C256-28DIP: IC EEPROM 256KBIT 150NS 28DIP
